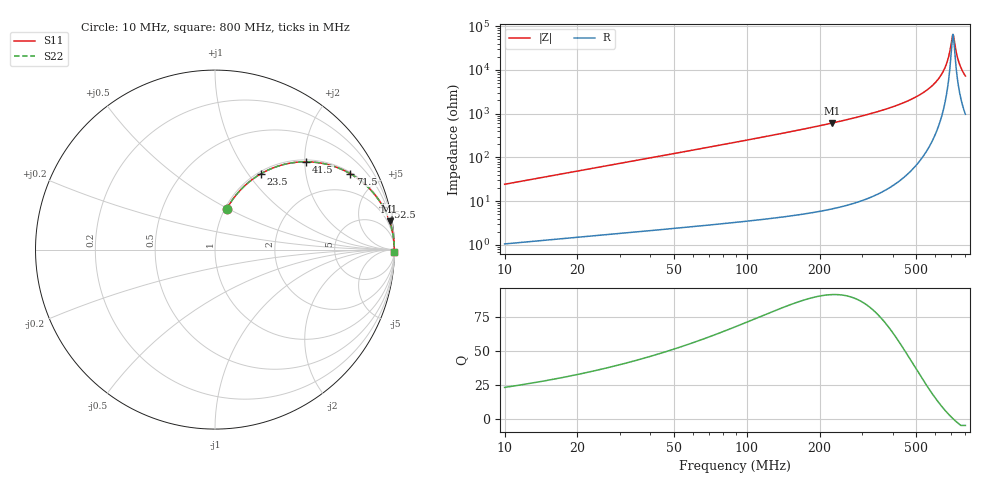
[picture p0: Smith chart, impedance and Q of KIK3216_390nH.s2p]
!version-2
!date-01.2022
!Series
# MHz S RI R 50
!Freq ReS11 ImS11 ReS21 ImS21 ReS12 ImS12 ReS22 ImS22
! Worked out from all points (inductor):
!   528 points, 10 MHz to 800 MHz, reference 50 ohm
!   read as one part in series: L = 388 nH near 13 MHz
!   highest Q = 91.4 at 226 MHz (marker M1), where L = 432 nH
!   self-resonance near 710.5 MHz
!   S11 on the Smith chart (normalised r, x): 10 MHz: 1.02, +0.49; 23.5 MHz: 1.03, +1.15; 41.5 MHz: 1.04, +2.03; 71.5 MHz: 1.06, +3.52; 152.5 MHz: 1.09, +7.79; 800 MHz: open
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10  0.0649 0.2256  0.9351 -0.2256  0.9351 -0.2256  0.0649 0.2256
23.5  0.2537 0.4212  0.7463 -0.4212  0.7463 -0.4212  0.2537 0.4212
41.5  0.5075 0.4894  0.4925 -0.4894  0.4925 -0.4894  0.5075 0.4894
71.5  0.7526 0.4233  0.2474 -0.4233  0.2474 -0.4233  0.7526 0.4233
101.5  0.8611 0.339  0.1389 -0.339  0.1389 -0.339  0.8611 0.339
142  0.9259 0.2559  0.0741 -0.2559  0.0741 -0.2559  0.9259 0.2559
152.5  0.9357 0.2393  0.0643 -0.2393  0.0643 -0.2393  0.9357 0.2393
226  0.9724 0.1584  0.0276 -0.1584  0.0276 -0.1584  0.9724 0.1584
274  0.9827 0.1251  0.0173 -0.1251  0.0173 -0.1251  0.9827 0.1251
406  0.9943 0.0676  0.00569 -0.0676  0.00569 -0.0676  0.9943 0.0676
538  0.9978 0.0325  0.00222 -0.0325  0.00222 -0.0325  0.9978 0.0325
617.5  0.9984 0.0162  0.00158 -0.0162  0.00158 -0.0162  0.9984 0.0162
646  0.9985 0.011  0.0015 -0.011  0.0015 -0.011  0.9985 0.011
668.5  0.9985 0.00707  0.00148 -0.00707  0.00148 -0.00707  0.9985 0.00707
686.5  0.9985 0.00401  0.0015 -0.00401  0.0015 -0.00401  0.9985 0.00401
706  0.9985 0.000787  0.00154 -0.000787  0.00154 -0.000787  0.9985 0.000787
710.5  0.9985 5.67e-05  0.00155 -5.67e-05  0.00155 -5.67e-05  0.9985 5.67e-05
716.5  0.9984 -0.00091  0.00157 0.00091  0.00157 0.00091  0.9984 -0.00091
734.5  0.9984 -0.00376  0.00163 0.00376  0.00163 0.00376  0.9984 -0.00376
749.5  0.9983 -0.00609  0.0017 0.00609  0.0017 0.00609  0.9983 -0.00609
772  0.9982 -0.0095  0.00183 0.0095  0.00183 0.0095  0.9982 -0.0095
800  0.998 -0.0136  0.00202 0.0136  0.00202 0.0136  0.998 -0.0136
